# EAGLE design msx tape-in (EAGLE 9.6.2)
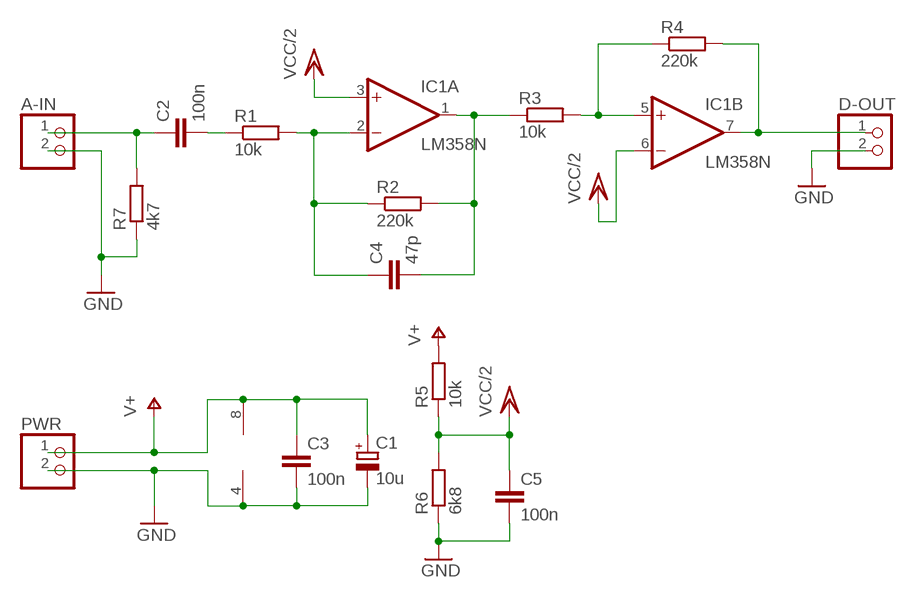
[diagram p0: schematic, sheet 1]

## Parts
A-IN  PINHD-1X2  [1X02]
C1  10u  CPOL-EUE2.5-5  [E2,5-5]
C2  100n  C-EU025-025X050  [C025-025X050]
C3  100n  C-EU025-025X050  [C025-025X050]
C4  47p  C-EU025-025X050  [C025-025X050]
C5  100n  C-EU025-025X050  [C025-025X050]
D-OUT  PINHD-1X2  [1X02]
IC1  LM358N  [DIL08]
PWR  PINHD-1X2  [1X02]
R1  10k  R-EU_0207/10  [0207/10]
R2  220k  R-EU_0207/10  [0207/10]
R3  10k  R-EU_0207/10  [0207/10]
R4  220k  R-EU_0207/10  [0207/10]
R5  10k  R-EU_0207/10  [0207/10]
R6  6k8  R-EU_0207/10  [0207/10]
R7  4k7  R-EU_0207/10  [0207/10]

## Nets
GND: A-IN.2 C1.- C3.2 C5.2 D-OUT.2 IC1.4(P:V-) PWR.2 R6.1 R7.1
N$1: C4.1 IC1.2(A:-IN) R1.2 R2.1
N$2: C2.2 R1.1
N$4: IC1.5(B:+IN) R3.2 R4.1
N$5: D-OUT.1 IC1.7(B:OUT) R4.2
N$6: A-IN.1 C2.1 R7.2
N$8: C4.2 IC1.1(A:OUT) R2.2 R3.1
V+: C1.+ C3.1 IC1.8(P:V+) PWR.1 R5.2
VCC/2: C5.1 IC1.3(A:+IN) IC1.6(B:-IN) R5.1 R6.2

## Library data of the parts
A-IN D-OUT PWR = pinhead:PINHD-1X2: PIN HEADER
C1 = rcl:CPOL-EU: POLARIZED CAPACITOR, European symbol; SPICEPREFIX: C
C2-C5 = rcl:C-EU: CAPACITOR, European symbol; SPICEPREFIX: C
IC1 = linear:LM358: OP AMP also LM158; LM258; LM2904 Source: http://cache.national.com/ds/LM/LM158.pdf
R1-R7 = rcl:R-EU_: RESISTOR, European symbol; SPICEPREFIX: R

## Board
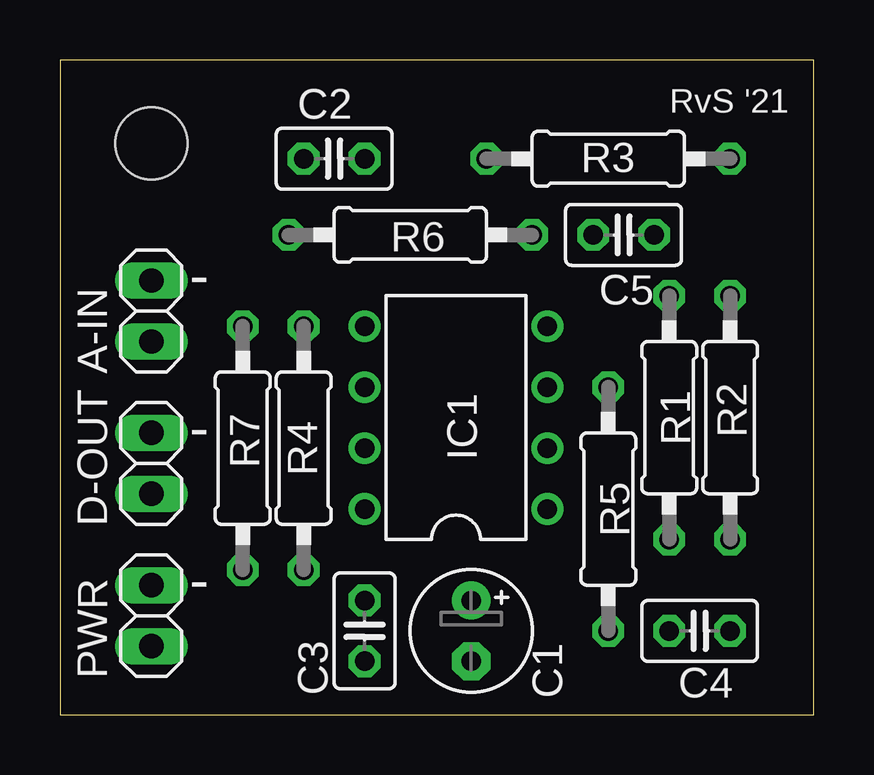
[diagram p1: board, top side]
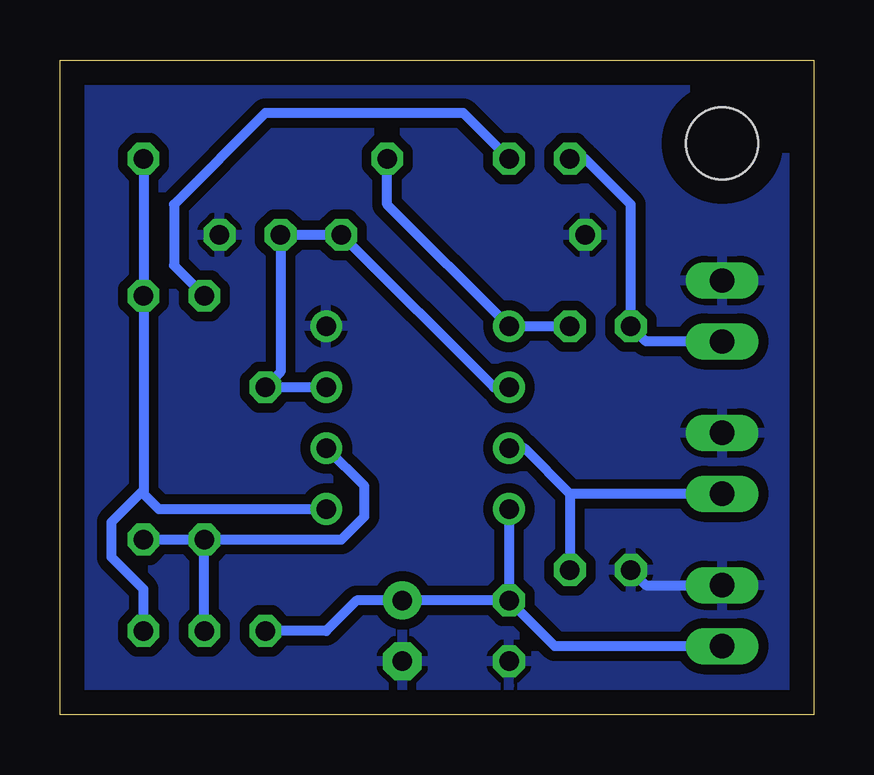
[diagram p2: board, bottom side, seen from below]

Size 31.42 x 27.3 mm. Coordinates in mm from the lower left corner, seen from the top.
Outline: 0,0 31.42,0 31.42,27.3 0,27.3 0,0
Copper layers 1*16: Top 0mil / dielectric 1.5mm / Bottom 0.035mm
Design rules "default *": minimum track width 6mil, minimum drill 0.35mm, track to track 6mil, track to pad 6mil, pad to pad 6mil, via to via 6mil, smd to smd 6mil, copper to edge 40mil, drill to drill 6mil, minimum pad ring 10mil, minimum via ring 8mil, stop-mask expansion 4mil, vias tented up to drill 0mil, thermal gap 10mil
Holes 3 mm at 3.81,23.81

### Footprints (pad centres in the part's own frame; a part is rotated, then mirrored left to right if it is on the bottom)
1X02 = drill 1.016 long: 1 -1.27,0; 2 1.27,0
E2,5-5 = drill 0.813 pad 1.6: + -1.27,0 | drill 0.813 pad 1.6 octagon: - 1.27,0
C025-025X050 = drill 0.813 octagon: 1 -1.27,0; 2 1.27,0
DIL08 = drill 0.813 pad 1.27: 1 -3.81,-3.81; 2 -1.27,-3.81; 3 1.27,-3.81; 4 3.81,-3.81; 5 3.81,3.81; 6 1.27,3.81; 7 -1.27,3.81; 8 -3.81,3.81
0207/10 = drill 0.813 octagon: 1 -5.08,0; 2 5.08,0

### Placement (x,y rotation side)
A-IN  3.81,16.83 90 top
C1  17.14,3.49 270 top
C2  11.43,23.18 0 top
C3  12.7,3.49 270 top
C4  26.67,3.49 0 top
C5  23.5,20 0 top
D-OUT  3.81,10.48 90 top
IC1  16.51,12.38 90 top
PWR  3.81,4.13 90 top
R1  25.4,12.38 270 top
R2  27.94,12.38 90 top
R3  22.86,23.18 180 top
R4  10.16,11.11 270 top
R5  22.86,8.57 270 top
R6  14.61,20 0 top
R7  7.62,11.11 90 top

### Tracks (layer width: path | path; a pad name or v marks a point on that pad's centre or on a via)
GND
  Bottom 0.406: R7.1 6.99,5.4 PWR.2
  pour Bottom (isolate 0.406): 0.32,0.95 31.11,0.95 31.11,26.35 0.32,26.35
N$1
  Bottom 0.406: R2.1 R1.2 | C4.1 R1.2 | IC1.2 18.73,9.53 18.73,8.25 19.68,7.3 R1.2
N$2
  Bottom 0.406: C2.2 14.61,25.08 22.86,25.08 26.67,21.27 26.67,18.73 R1.1
N$4
  Bottom 0.406: R4.1 IC1.5 17.78,21.27 R3.2
N$5
  Bottom 0.406: D-OUT.1 10.16,9.21 | 10.16,9.21 12.06,11.11 IC1.7 | 10.16,9.21 R4.2
N$6
  Bottom 0.406: C2.1 9.53,23.18 7.62,21.27 R7.2 6.99,15.56 A-IN.1
N$8
  Bottom 0.406: 27.94,9.36 R2.2 R3.1 | C4.2 27.94,5.23 29.27,6.56 29.27,8.03 27.94,9.36 | 27.94,9.36 27.94,9.21 27.3,8.57 IC1.1
V+
  Bottom 0.406: IC1.8 C3.1 | C3.1 C1.+ 19.05,4.76 20.32,3.49 R5.2 | PWR.1 10.79,2.86 C3.1
VCC/2
  Bottom 0.406: IC1.3 R5.1 22.23,14.29 C5.1 R6.2 13.34,13.65 IC1.6

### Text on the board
tNames: RvS '21 | - | - | -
